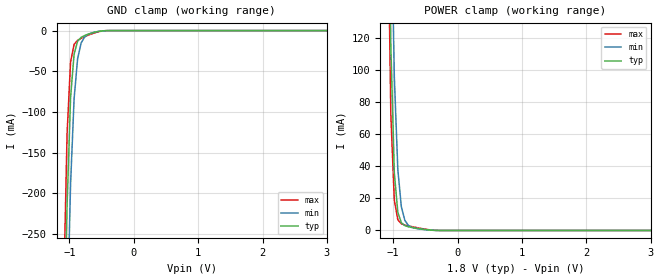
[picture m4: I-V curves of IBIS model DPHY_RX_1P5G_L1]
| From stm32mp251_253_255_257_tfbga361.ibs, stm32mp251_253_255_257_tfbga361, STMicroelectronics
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[Model] DPHY_RX_1P5G_L1
Model_type   Input
Polarity   Non-Inverting
Enable   Active-High
C_comp   0.873pF   0.86pF   0.89pF
Vinh = 460.000mV
Vinl = -40.000mV
[Model Spec]
[Temperature Range]   25.000   -40.000   125.000
[Voltage Range]   1.800V   1.516V   2.030V
[GND Clamp Reference]   0.00V   0.00V   0.00V
[POWER Clamp Reference]   1.800V   1.516V   2.030V
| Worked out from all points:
|   GND clamp passes 1 mA (typ) near -0.55 V on its own axis
|   POWER clamp passes 1 mA (typ) near -0.58 V on its own axis
[GND Clamp]
-1.8V     -4.02A     -4.056A    -4.004A
-1.091V   -434mA     -593.6mA   -327.1mA
-1.036V   -215mA     -362.6mA   -126.7mA
-981.8mV  -82.23mA   -188.9mA   -38.51mA
-927.3mV  -28.93mA   -84.03mA   -16.99mA
-872.7mV  -13.17mA   -34.74mA   -11.93mA
-818.2mV  -8.3mA     -15.29mA   -9.536mA
-763.6mV  -6.035mA   -7.844mA   -7.569mA
-709.1mV  -4.42mA    -4.64mA    -5.742mA
-600mV    -1.904mA   -1.792mA   -2.573mA
-436.4mV  -95.62uA   -166.9uA   -107.1uA
3.545V    250.5nA    800.3nA    1.158uA
[Power Clamp]
-1.745V   4.14A      4.118A     4.251A
-1.091V   293.3mA    412.5mA    225.2mA
-1.036V   114.9mA    215.6mA    72.01mA
-981.8mV  35.72mA    95.68mA    18.8mA
-927.3mV  11.28mA    37.9mA     6.643mA
-872.7mV  4.836mA    14.76mA    4.171mA
-818.2mV  3.015mA    6.287mA    3.374mA
-763.6mV  2.298mA    3.192mA    2.849mA
-654.5mV  1.472mA    1.36mA     1.931mA
-436.4mV  295.6uA    287.6uA    422.2uA
-218.2mV  792.2nA    4.408uA    980.9nA
3.6V      -29.89nA   -214.4nA   -70.43nA
